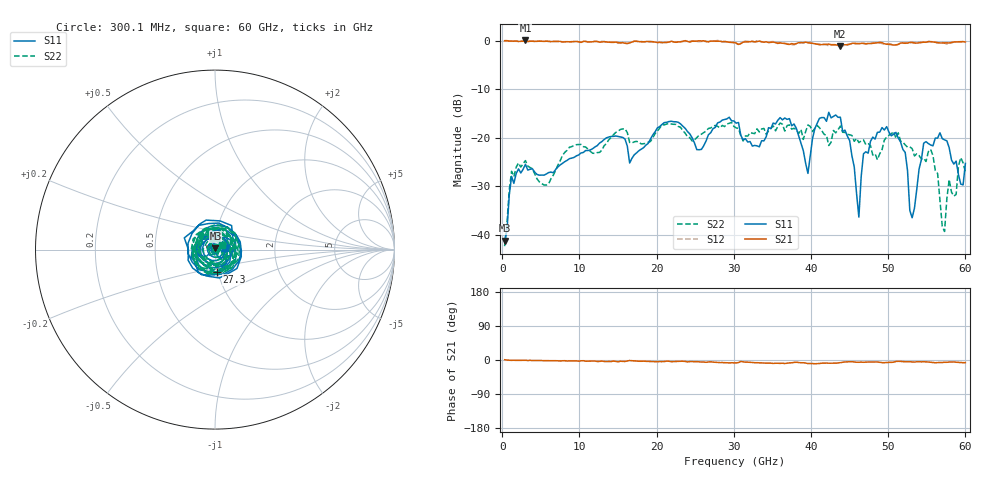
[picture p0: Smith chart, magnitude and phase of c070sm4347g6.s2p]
! 3/17/2022 10:11:49 AM
! D:\C070SM4347G6.S2P
! CHANNEL.1
! TR.MEASUREMENT
! CORRECTED.DATA
# GHZ S RI R 50.0
! FREQ.GHZ  S11RE  S11IM  S21RE  S21IM  S12RE  S12IM  S22RE  S22IM
!; PortSelection: Port_12
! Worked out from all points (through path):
!   200 points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, 300.1 MHz to 60 GHz, reference 50 ohm
!   highest |S21| = 0.02 dB at 3 GHz (marker M1); lowest = -1.1 dB at 43.8 GHz (marker M2)
!   lowest |S11| = -41.2 dB at 300.1 MHz (marker M3), VSWR 1.02, Z = 50.3 + j0.838 ohm
!   |S11| at or under -10 dB: start of sweep to end of sweep
!   |S22| runs from -42.3 to -16.8 dB; largest |S21 - S12| = 0.041
!   S11 on the Smith chart (normalised r, x): 300.1 MHz: 1.01, +0.02; 27.3 GHz: 0.99, -0.25; 60 GHz: 1.11, +0.02
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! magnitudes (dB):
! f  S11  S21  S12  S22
! 300.1 MHz  -41.2  0.0  0.0  -42.3
! 1.2 GHz  -27.9  -0.1  -0.1  -26.9
! 3 GHz  -25.5  0.0  0.0  -24.7
! 5.7 GHz  -27.5  -0.1  -0.1  -29.7
! 10.5 GHz  -23.0  -0.2  -0.2  -21.8
! 20.4 GHz  -17.7  -0.3  -0.4  -18.0
! 27.3 GHz  -18.1  -0.1  -0.1  -17.6
! 30.3 GHz  -17.0  -0.5  -0.7  -18.0
! 37.2 GHz  -16.1  -0.8  -0.8  -17.3
! 39.6 GHz  -27.3  -0.4  -0.4  -17.4
! 40.2 GHz  -20.1  -0.6  -0.5  -18.7
! 43.8 GHz  -15.8  -1.1  -1.2  -17.6
! 46.2 GHz  -36.3  -0.6  -0.6  -21.0
! 46.8 GHz  -23.3  -0.6  -0.6  -20.4
! 50.1 GHz  -18.8  -0.8  -0.6  -19.5
! 52.2 GHz  -23.0  -0.6  -0.4  -21.5
! 53.1 GHz  -36.5  -0.4  -0.4  -22.2
! 54.6 GHz  -21.1  -0.3  -0.3  -24.2
! 55.8 GHz  -21.7  -0.3  -0.2  -23.7
! 57.3 GHz  -20.4  -0.5  -0.5  -39.3
! 57.9 GHz  -22.0  -0.5  -0.6  -28.6
! 60 GHz  -25.3  -0.3  -0.2  -27.0
